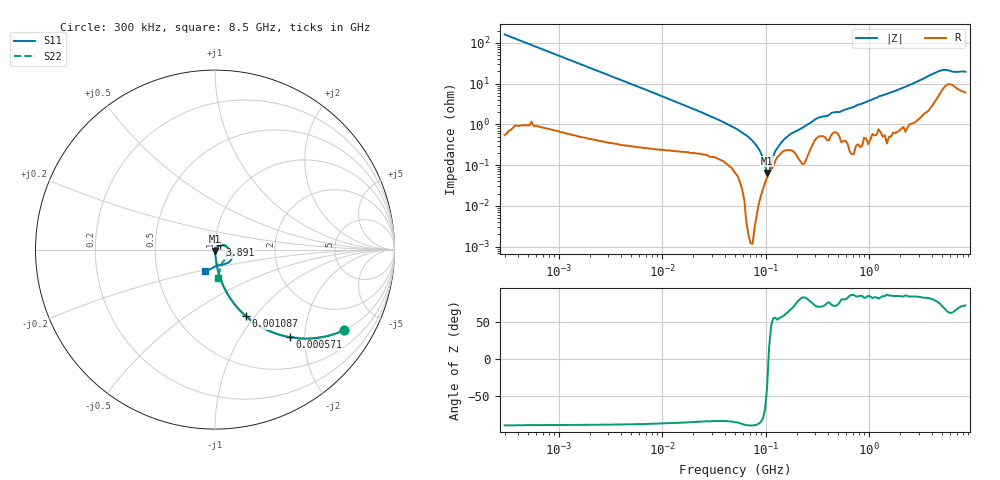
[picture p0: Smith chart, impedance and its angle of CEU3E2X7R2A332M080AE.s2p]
! S-parameter Generated by TDK Corporation
! Copyright(C) 2015 TDK Corporation.
! All Rights Reserved.
! TDK P/N: CEU3E2X7R2A332M080AE (Multilayer Ceramic Chip Capacitors)
! Property: C=3.3nF
! Size(LxWxT): 1.6x0.8x0.8mm, 0.063x0.031x0.031inches
! Model Type: s2p (Touchstone File Format Version 1.0)
! Frequency: DC=Yes Start=0.3MHz Stop=8500MHz 225points Log-sweep
! Note:
! Model Generated on Jun. 23, 2015
! Hash(MD5):
! Port Assignments:
!  1 ---| |--- 2
! Applicable Conditions:
!  Temperature = 25 degC
!  DC Bias Voltage = 0 V
!  Small Signal Operation
! Terms and conditions regarding TDK Simulation Models
! (1)This simulation model is being provided solely for informational purposes. Please refer to the specifications of the products in terms of detailed characteristics of such products.
! (2)In no event shall TDK Corporation of any of its subsidiaries be liable for any loss or damage arising, directly or indirectly,
!  From any information contained in this simulation model, including, but not limited to loss or damages arising from any inaccuracies, omissions or errors in connection with such information.
! (3)Any and all copyrights on this simulation model are owned by TDK Corporation.
!  Duplication or redistribution of this simulation model without prior written permission from TDK Corporation is prohibited.
! (4)This simulation model is subject to any modification or change without any prior notice.
! (5)Neither TDK Corporation nor any of its subsidiaries shall make any warranty, express or implied,
!  Including but not limited to the correctness, implied warranties of merchantability and fitness for a particular purpose with respect to this simulation models.
! (6)The use of this simulation model shall be deemed to have consented to the terms and conditions hereof.
# MHz S MA R 50
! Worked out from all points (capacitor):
!   224 points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, 300 kHz to 8.5 GHz, reference 50 ohm
!   read as one part in series: C = 3.29 nF near 314.1 kHz
!   lowest |Z| = 64 mohm at 103 MHz (marker M1)
!   series resonance near 106.4 MHz, so ESL is about 680 pH
!   S11 on the Smith chart (normalised r, x): 300 kHz: 1.00, -3.21; 571 kHz: 1.02, -1.69; 1.087 MHz: 1.01, -0.90; 3.891 GHz: 1.05, +0.05; 8.5 GHz: 0.87, -0.21
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0.3  0.8484 -31.9  0.5275 57.9  0.5286 58.1  0.8479 -31.9
0.5710021  0.6432 -49.4  0.7577 40.0  0.7582 40.1  0.643 -49.4
1.086811  0.4072 -65.2  0.9076 24.0  0.9076 24.1  0.4069 -65.2
1.72111  0.2722 -73.3  0.9576 15.8  0.9577 15.8  0.2721 -73.3
9.430415  0.05201 -84.9  0.9959 2.9  0.9964 3.0  0.05238 -84.3
51.67171  0.009366 -101.5  0.9976 0.3  0.998 0.3  0.01144 -89.4
102.9757  0.007569 -108.3  0.9968 -0.3  0.9972 -0.2  0.003255 -119.7
148.7505  0.003995 -56.8  0.9961 -0.5  0.9966 -0.5  0.0008125 154.3
205.2186  0.0009993 -67.2  0.9966 -0.8  0.9972 -0.8  0.00139 111.4
283.1228  0.003967 -24.5  0.9954 -1.2  0.9959 -1.2  0.006283 89.0
491.5417  0.007572 48.4  0.9931 -2.1  0.9937 -2.0  0.006514 -10.8
678.1388  0.004454 123.9  0.9941 -2.9  0.9948 -2.9  0.001246 -150.2
743.4462  0.001387 78.1  0.9941 -3.2  0.9948 -3.1  0.002397 75.1
893.5346  0.003476 -29.2  0.9938 -3.8  0.994 -3.7  0.006001 50.3
979.5854  0.00214 78.6  0.9938 -4.2  0.9947 -4.1  0.002447 53.0
1290.729  0.01033 56.7  0.9926 -5.4  0.9931 -5.4  0.006333 -3.4
1481.602  0.005016 87.6  0.9926 -6.3  0.9931 -6.2  0.002284 88.3
1551.304  0.003276 67.1  0.9917 -6.5  0.9923 -6.5  0.004414 43.6
1624.285  0.001701 37.8  0.9913 -6.8  0.9922 -6.8  0.004804 53.8
1864.484  0.00583 18.3  0.9907 -7.8  0.9914 -7.8  0.003646 26.6
3890.506  0.03634 41.7  0.9717 -16.8  0.972 -16.7  0.03985 35.3
8500  0.1324 -114.1  0.9186 -31.0  0.9199 -31.1  0.1616 -84.9
